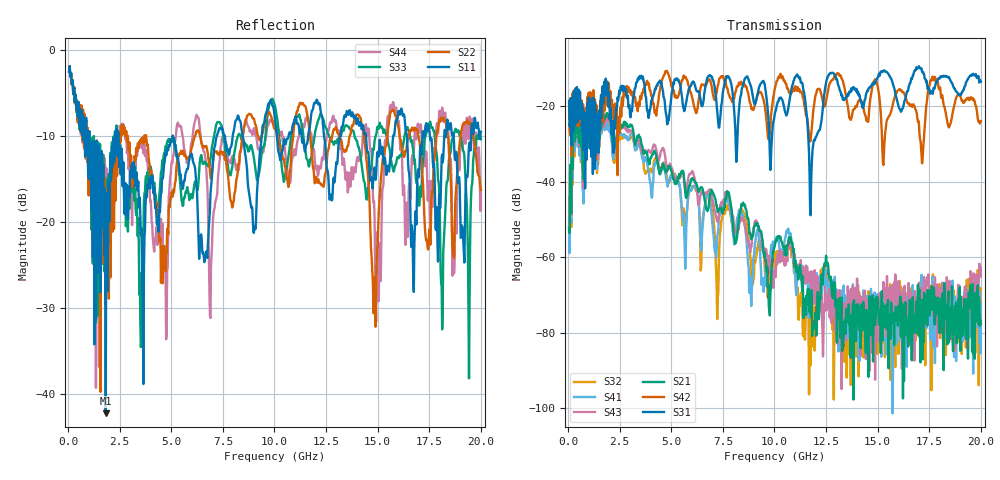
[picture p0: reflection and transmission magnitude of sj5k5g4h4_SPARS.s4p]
! FILE: E:\users\goganessyan\GBX_Backplane\FR408_backplane\1m_OUTBOUND_FEXT\sj5k5g4h4_SPARS.s4p
# MHZ S RI R 50.00
! FREQ  S11  S12  S13  S14
!  S21  S22  S23  S24
!  S31  S32  S33  S34
!  S41  S42  S43  S44
!  REAL  IMAG  REAL  IMAG  REAL  IMAG  REAL  IMAG
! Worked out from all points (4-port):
!   799 points, 50 MHz to 20 GHz, reference 50 ohm
!   strongest paths, dB at 50 MHz, 5.025 GHz, 10.03 GHz, 15.03 GHz, 20 GHz:
!     S31: -18.6, -16.3, -21.7, -12.2, -13.5
!     S42: -19.3, -14.9, -15.1, -15.4, -24.0
!     S21: -52.5, -37.6, -56.6, -72.4, -77.6
!     S43: -52.8, -36.5, -63.0, -82.3, -65.1
!     S41: -51.0, -39.0, -56.2, -70.0, -72.4
!     S32: -52.1, -38.1, -59.4, -73.2, -77.8
!   lowest |S11| = -42.2 dB at 1.825 GHz (marker M1), VSWR 1.02, Z = 50.7 - j0.292 ohm
!   |S11| at or under -10 dB: 2.435 GHz to 5.066 GHz (2.631 GHz wide, 70.2 % of centre); 5.078 GHz to 7.203 GHz (2.124 GHz wide, 34.6 % of centre); 14.43 GHz to 15.75 GHz (1.319 GHz wide, 8.74 % of centre)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
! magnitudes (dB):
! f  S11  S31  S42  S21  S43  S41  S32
! 50 MHz  -2.5  -18.6  -19.3  -52.5  -52.8  -51.0  -52.1
! 1.825 GHz  -42.2  -12.7  -14.3  -22.9  -24.2  -26.0  -25.0
! 6.85 GHz  -19.5  -11.8  -12.9  -44.5  -42.6  -44.0  -42.5
! 7.225 GHz  -9.9  -21.3  -15.3  -47.1  -50.6  -54.4  -76.4
! 11.75 GHz  -8.1  -48.9  -29.1  -70.9  -66.9  -66.3  -88.6
! 12.72 GHz  -16.8  -11.2  -13.5  -65.2  -76.4  -75.2  -70.9
! 20 GHz  -9.5  -13.5  -24.0  -77.6  -65.1  -72.4  -77.8
